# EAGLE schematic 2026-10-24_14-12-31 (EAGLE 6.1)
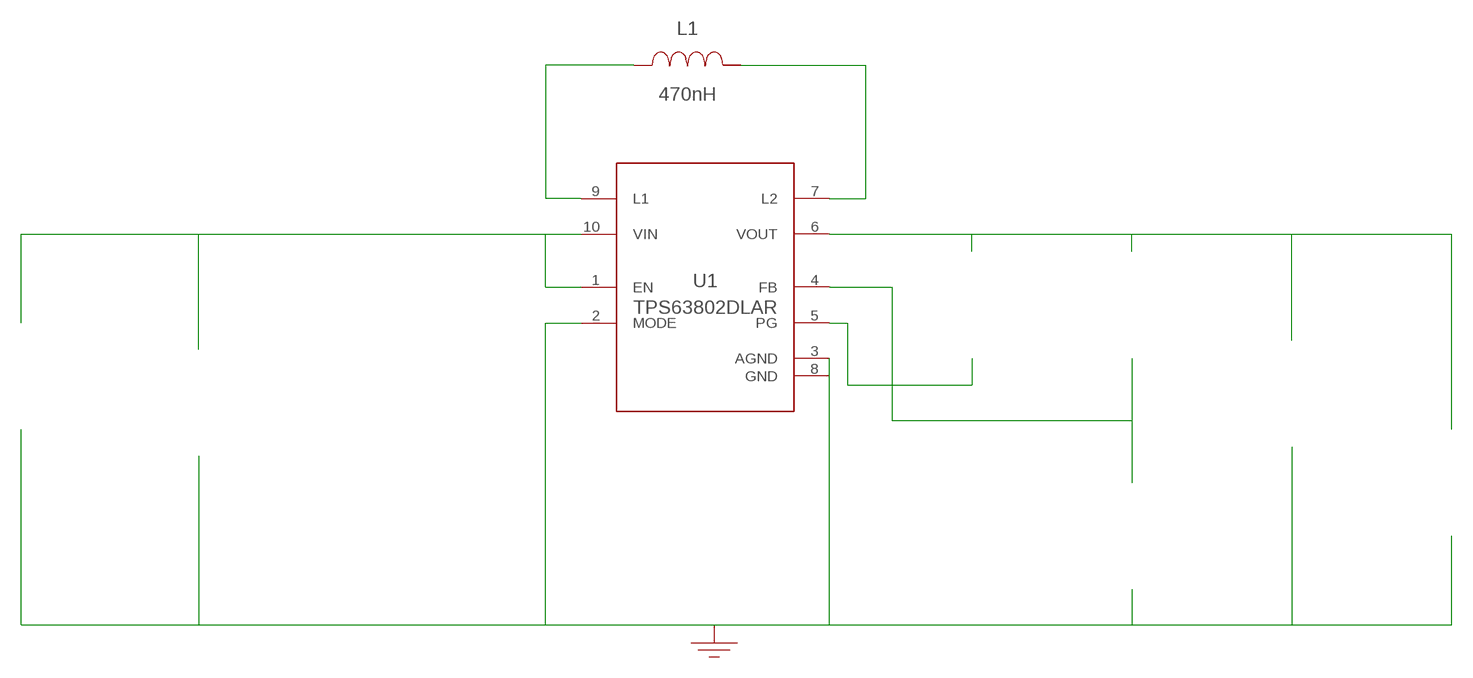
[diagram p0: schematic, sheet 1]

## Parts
CIN  22uF  GRM188R60J226MEA0DGRM188R60J226MEA0D  [0603]  (not placed on a sheet)
COUT  22uF  MSASL219LB5226MTNA01MSASL219LB5226MTNA01  [0805]  (not placed on a sheet)
GND  WB_GND  WB_GNDWB_GND  [WB_GND]
IOUT  WB_CURRENT_LOAD  WB_CURRENT_LOADWB_CURRENT_LOAD  [WB_CURRENT_LOAD]  (not placed on a sheet)
L1  470nH  XFL4015-471MEBXFL4015-471MEB  [XFL4015]
RFBB  91k  RC0603FR-0791KLRC0603FR-0791KL  [0603]  (not placed on a sheet)
RFBT  511k  CRCW0402511KFKEDCRCW0402511KFKED  [0402]  (not placed on a sheet)
RPG  100k  CRCW0402100KFKEDCRCW0402100KFKED  [0402]  (not placed on a sheet)
U1  TPS63802DLAR  TPS63802DLARTPS63802DLAR  [DLA0010A]
VIN  WB_BATTERY  WB_BATTERYWB_BATTERY  [WB_BATTERY]  (not placed on a sheet)
Unconnected: CIN.1 CIN.2 COUT.1 COUT.2 GND.1 IOUT.1(+) IOUT.2(-) L1.1 L1.2 RFBB.1 RFBB.2 RFBT.1 RFBT.2 RPG.1 RPG.2 U1.1(EN) U1.2(MODE) U1.4(FB) U1.5(PG) U1.7(L2) U1.9(L1) VIN.1(+) VIN.2(-)

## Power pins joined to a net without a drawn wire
AGND: U1.3(AGND)
GND: U1.8(GND)
VIN: U1.10(VIN)
VOUT: U1.6(VOUT)

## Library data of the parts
CIN = AcceleratedDesigns_Lib:GRM188R60J226MEA0D; Manufacturer_Part_Number: GRM188R60J226MEA0D; Vendor: MuRata
COUT = AcceleratedDesigns_Lib:MSASL219LB5226MTNA01; Manufacturer_Part_Number: MSASL219LB5226MTNA01; Vendor: Taiyo Yuden
GND = AcceleratedDesigns_Lib:WB_GND; Manufacturer_Part_Number: WB_GND
IOUT = AcceleratedDesigns_Lib:WB_CURRENT_LOAD; Manufacturer_Part_Number: WB_CURRENT_LOAD
L1 = AcceleratedDesigns_Lib:XFL4015-471MEB; Manufacturer_Part_Number: 'XFL4015-471MEB'; Vendor: Gimme a name
RFBB = AcceleratedDesigns_Lib:RC0603FR-0791KL; Manufacturer_Part_Number: RC0603FR-0791KL; Vendor: Yageo America
RFBT = AcceleratedDesigns_Lib:CRCW0402511KFKED; Manufacturer_Part_Number: CRCW0402511KFKED; Vendor: Vishay-Dale
RPG = AcceleratedDesigns_Lib:CRCW0402100KFKED; Manufacturer_Part_Number: CRCW0402100KFKED; Vendor: Vishay-Dale
U1 = AcceleratedDesigns_Lib:TPS63802DLAR; Manufacturer_Part_Number: TPS63802DLAR
VIN = AcceleratedDesigns_Lib:WB_BATTERY; Manufacturer_Part_Number: WB_BATTERY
